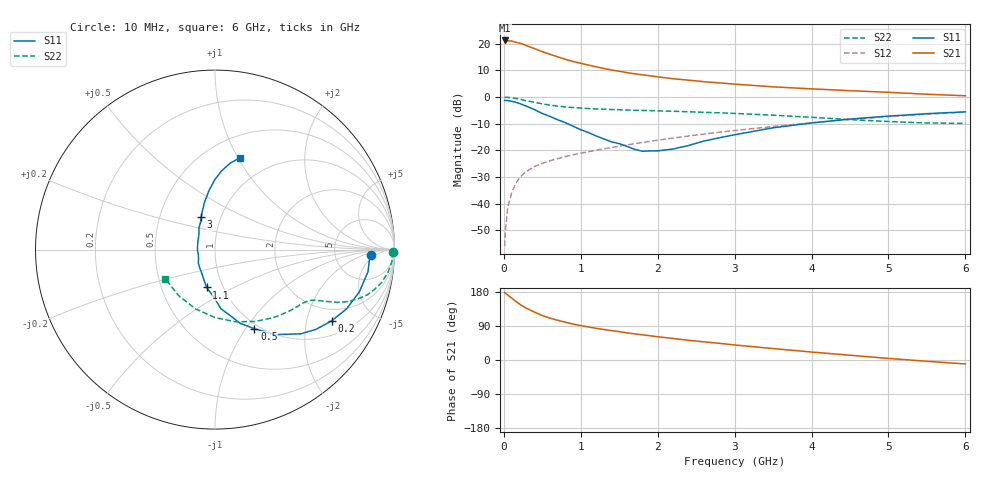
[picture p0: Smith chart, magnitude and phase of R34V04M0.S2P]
! SIEMENS Small Signal Semiconductors
! BFR181
! Si NPN RF Bipolar Junction Transistor in SOT23
! VCE = 4 V  IC = 4 mA
! Common Emitter S-Parameters:  May  1996
# GHz  S  MA  R  50
!  f  S11  S21  S12  S22
! GHz  MAG  ANG  MAG  ANG  MAG  ANG  MAG  ANG
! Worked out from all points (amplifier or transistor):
!   36 points, 10 MHz to 6 GHz, reference 50 ohm
!   highest |S21| = 21.2 dB at 10 MHz (marker M1)
!   |S21| within 3 dB of that: start of sweep to 392.7 MHz
!   unconditionally stable (mu >= 1): 1.241 GHz to 3.077 GHz
!   at 250 MHz: K = 0.36, MSG = 24.4 dB, |S12| = -28.9 dB
!   at 1.4 GHz: K = 1.03, MAG = 13.4 dB, |S12| = -18.9 dB
!   at 6 GHz: K = 0.86, MSG = 3.1 dB, |S12| = -5.6 dB
!   S11 on the Smith chart (normalised r, x): 10 MHz: 13, -3; 200 MHz: 1.50, -2.84; 500 MHz: 0.94, -1.10; 1.1 GHz: 0.84, -0.37; 3 GHz: 0.80, +0.30; 6 GHz: 0.72, +1.02
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0.01  0.8674 -1.9  11.54 178.2  0.0016 87.8  0.9936 -0.8
0.02  0.8629 -3.1  11.28 176.4  0.003 88.5  0.9884 -1.6
0.05  0.8614 -8.2  11.35 171.7  0.0084 84.9  0.9882 -3.9
0.1  0.8377 -16.4  11.24 163.8  0.0158 80.9  0.9716 -7.6
0.15  0.8041 -24.2  10.7 155.4  0.0233 76.7  0.9474 -11.1
0.2  0.7619 -31.4  10.33 148.4  0.03 73.5  0.9172 -13.9
0.25  0.7161 -38.4  9.815 141.6  0.0357 70.1  0.8845 -16.6
0.3  0.6695 -44.5  9.159 135.9  0.0408 68.1  0.8516 -18.5
0.4  0.5807 -54.6  8.095 126.3  0.0501 64.6  0.7975 -21.3
0.5  0.4929 -63.5  7.118 117.3  0.0573 62.9  0.7462 -23.2
0.6  0.4333 -71.2  6.353 110.5  0.064 61.8  0.7063 -24.3
0.8  0.331 -84.3  5.111 99.6  0.0766 60.7  0.655 -25.8
0.9  0.2846 -88.9  4.661 94.9  0.0828 61.0  0.6378 -26.4
1.1  0.2162 -102.4  3.985 87.2  0.0946 61.6  0.6098 -27.6
1.3  0.1642 -114.3  3.444 80.5  0.1074 62.1  0.5913 -29.0
1.6  0.1192 -141.4  2.878 71.7  0.1272 62.4  0.5725 -31.5
2.2  0.1062 153.4  2.212 56.8  0.1705 61.4  0.5425 -38.4
3  0.1967 113.3  1.749 39.7  0.2362 57.6  0.4938 -50.6
3.5  0.2657 103.1  1.558 30.2  0.2807 53.9  0.4578 -61.0
4.5  0.3871 90.4  1.318 12.6  0.3797 44.1  0.3784 -90.0
5.5  0.4886 80.1  1.132 -3.4  0.4769 31.6  0.327 -128.2
6  0.529 75.0  1.058 -10.4  0.5219 24.6  0.3208 -149.4
